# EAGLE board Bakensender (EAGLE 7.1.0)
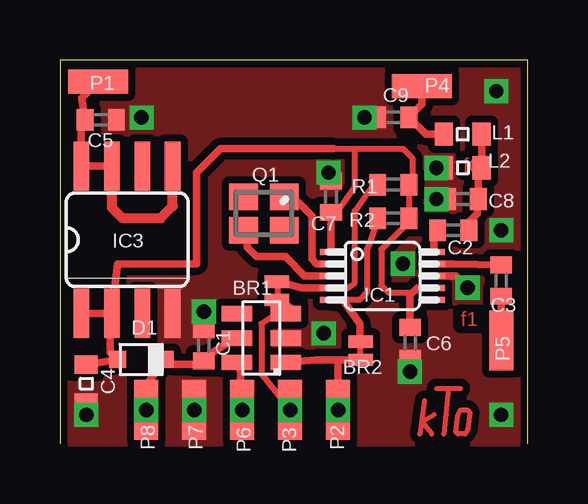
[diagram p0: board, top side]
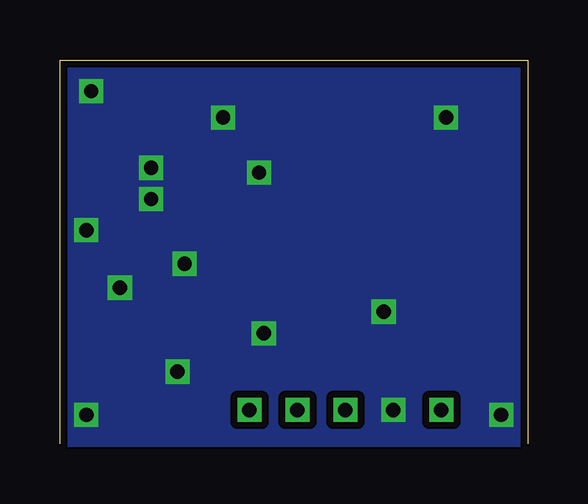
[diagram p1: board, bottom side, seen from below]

Size 19.5 x 16 mm. Coordinates in mm from the lower left corner, seen from the top.
Outline: 19.5,0 19.5,16 0,16 0,0
Copper layers (1*16): Top 0.035mm / dielectric 0.5mm / Bottom 0.035mm
Design rules "default *": minimum track width 10mil, minimum drill 0.6mm, track to track 8mil, track to pad 8mil, pad to pad 8mil, via to via 8mil, smd to smd 8mil, copper to edge 4mil, drill to drill 8mil, minimum pad ring 10mil, minimum via ring 8mil, stop-mask expansion 4mil, vias tented up to drill 0mil, thermal gap 10mil

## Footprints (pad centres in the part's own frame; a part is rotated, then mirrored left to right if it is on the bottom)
0402 = smd 0.7 x 0.9: 1 -0.65,0; 2 0.65,0
0603 = smd 0.762 x 0.965: 1 -0.787,0; 2 0.787,0
SOD323_S = smd 0.7 x 0.7: P$1 -0.997,-0.005; P$2 0.997,-0.005
MSOP10 = smd 0.25 x 0.9: 1 0,0; 2 0.5,0; 3 1,0; 4 1.5,0; 5 2,0; 6 2,4.3; 7 1.5,4.3; 8 1,4.3; 9 0.5,4.3; 10 0,4.3
SOT23-6 = smd 0.635 x 1.27: 1 -1.016,-1.016; 2 0,-1.016; 3 1.016,-1.016; 4 1.016,1.016; 5 0,1.016; 6 -1.016,1.016
SO08 = smd 0.66 x 2.032: 1 -1.905,-3.073; 2 -0.635,-3.073; 3 0.635,-3.073; 4 1.905,-3.073; 5 1.905,3.073; 6 0.635,3.073; 7 -0.635,3.073; 8 -1.905,3.073
ANSCHL7 = smd 2.5 x 1: P$1 0,0
FA-20H = smd 1.2 x 1.1: 1 -0.85,-0.7; 2 0.85,-0.7; 3 0.85,0.7; 4 -0.85,0.7
SMDJUMP = smd 1.016 x 0.508: P$1 0.051,0.508; P$2 0.051,-0.254

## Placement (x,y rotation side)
C1  100n  [0402]  6,4.1 90 top
C2  10n  [0402]  16.4,8.9 180 top
C3  10n  [0402]  18.4,6.8 90 top
C4  1u/6V  [0603]  1.1,2.5 90 top
C5  100n  [0402]  1.7,13.5 180 top
C6  100n  [0402]  14.6,4.2 90 top
C7  100n  [0402]  11.3,10.3 90 top
C8  39p  [0402]  16.8,10.2 0 top
C9  39p  [0402]  13.9,13.6 0 top
D1  BAT 62-03W  [SOD323_S]  3.4,3.5 180 top
IC1  SI5351A  [MSOP10]  11.3,8 270 top
IC2  PIC10F206  [SOT23-6]  8.4,4.4 90 top
IC3  MIC5200  [SO08]  2.8,8.5 0 top
L1  47nH  [0603]  16.8,12.9 180 top
L2  entfällt  [0603]  16.8,11.5 0 top
P1  +Ub  [ANSCHL7]  1.6,15.1 180 top
P2  Clk  [ANSCHL7]  11.6,1.4 270 top
P3  Data  [ANSCHL7]  9.6,1.4 270 top
P4  f0  [ANSCHL7]  15.1,14.9 0 top
P5  f1  [ANSCHL7]  18.4,4.3 270 top
P6  MCLR  [ANSCHL7]  7.6,1.4 270 top
P7  GND  [ANSCHL7]  5.6,1.4 270 top
P8  3V3  [ANSCHL7]  3.6,1.4 270 top
Q1  40MHz  [FA-20H]  8.5,9.6 180 top
R1  4k7  [0402]  13.9,10.8 0 top
R2  4k7  [0402]  13.9,9.4 0 top
U$9  SMDJUMP  [SMDJUMP]  12.6,4 180 top
U$10  SMDJUMP  [SMDJUMP]  9.1,6.5 180 top
U$11  [KTO]  15.6,1.1 0 top

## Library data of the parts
C1-C9 D1 IC3 R1 R2 = otto
IC1 = otto_afu
IC2 = microchip-3
L1 L2 P1-P8 U$9-U$11 = otto_L
Q1 = crystal

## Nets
GND: C1.2 C4.1 C5.1 C6.1 C7.2 C8.1 C9.1 IC1.8 IC2.2 IC3.4 L2.1 P7.P$1
N$1: IC2.1 P2.P$1 U$9.P$1
N$2: IC2.3 P3.P$1 U$10.P$1
N$3: IC1.3 Q1.3
N$4: IC1.2 Q1.1
N$5: IC2.6 P6.P$1
N$7: C3.1 P5.P$1
N$8: IC1.5 R2.1 U$9.P$2
N$9: C5.2 IC3.5 IC3.7 IC3.8 P1.P$1
N$10: C3.2 IC1.9
N$11: C2.2 IC1.10
N$12: C4.2 C6.2 C7.1 D1.P$2 IC1.1 IC1.7 IC3.1 IC3.2 R1.2 R2.2
N$14: IC1.4 R1.1 U$10.P$2
N$15: C1.1 D1.P$1 IC2.5 P8.P$1
N$16: C2.1 C8.2 L1.1 L2.2
N$17: C9.2 L1.2 P4.P$1

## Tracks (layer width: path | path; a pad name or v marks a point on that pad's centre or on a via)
GND  (via drill 0.6)
  Top 0.305: IC1.8 16.5,7 v17,6.5
  other vias: 18.2,14.7 6,5.5 11.2,11.3 14.6,3 14.3,7.5 18.4,1.2 11,4.6 1.1,1.2 3.4,13.6 5.6,1.4 12.7,13.6 15.7,10.2 15.7,11.5 18.4,8.9
  pour Top (isolate 0.305, no thermals): 0,16 19.5,16 19.5,0 0,0
  pour Bottom (isolate 0.305, no thermals): 0,16 19.5,16 19.5,0 0,0
N$1  (via drill 0.6)
  Top 0.305: IC2.1 10.7,3.48 11.6,3.48 | 11.6,3.48 12.3,3.48 12.31,3.49 U$9.P$1 | P2.P$1 11.6,3.48
  other vias: 11.6,1.4
N$2  (via drill 0.6)
  Top 0.254: 9.8,5.53 9.23,5.53 8.4,5 8.4,2.9 P3.P$1
  Top 0.305: IC2.3 9.8,5.53 9.89,5.53 U$10.P$1
  other vias: 9.6,1.4
N$3
  Top 0.305: IC1.3 10.2,7 9.4,7.8 8.2,7.8 7.8,8.2 7.8,8.75 Q1.3
N$4
  Top 0.305: IC1.2 10.7,7.5 10.5,7.7 10.5,9.5 9.9,10.1 9.55,10.1 Q1.1
N$5  (via drill 0.6)
  Top 0.305: P6.P$1 7.5,3.2 IC2.6
  other vias: 7.6,1.4
N$6
  Top 0.254: 12.5,4.2 12.5,3.6
N$7
  Top 0.305: C3.1 P5.P$1
N$8
  Top 0.254: R2.1 13.05,8.75 12.8,8.1 12.8,6.3 12.5,6 IC1.5
  Top 0.305: IC1.5 11.8,6 12.5,5 12.5,4.3 U$9.P$2
N$9
  Top 0.305: P1.P$1 0.91,14.41 C5.2 0.9,13.48 IC3.8 IC3.7
  Top 0.406: IC3.7 2.17,9.84 2.6,9.4 4.2,9.4 4.7,9.9 4.7,11.27 IC3.5
N$10
  Top 0.305: IC1.9 16.41,7.5 C3.2
N$11
  Top 0.305: IC1.10 15.6,8.79 C2.2
N$12
  Top 0.254: 11.4,12.3 12.3,12.3 | 12.3,12.3 14.3,12.3 14.7,11.9 14.7,10.65 R1.2 R2.2 14.5,9.2 13.4,8.1 13.4,6.6 13.7,6.3 14.5,6.3 14.6,6.2 14.65,6.25 | C7.1 11.35,9.35 12.3,10.7 12.3,12.3
  Top 0.305: 2.1,5.1 2.4,7.5 5.7,7.5 5.7,11.3 6.7,12.3 11.4,12.3 | IC1.1 C7.1 11.21,9.5 | C6.2 14.6,5.1 | IC1.7 14.9,6.5 14.6,6.2 14.6,5.1 | 14.6,5.1 14.5,5 | IC3.1 IC3.2 2.14,5.1 2.1,5.1 | C4.2 2.32,3.49 D1.P$2 2.1,3.81 2.1,5.1
N$14
  Top 0.254: IC1.4 12,6.5 12.3,6.7 12.3,9.7 13.2,11 R1.1
  Top 0.305: IC1.4 10.1,6.5 U$10.P$2
N$15  (via drill 0.6)
  Top 0.305: IC2.5 7.3,4.4 5.9,3.5 6.1,3.39 C1.1 5.85,3.3 4.8,3.3 4.61,3.4 D1.P$1 3.5,2.3 3.6,2.2 P8.P$1
  other vias: 3.6,1.4
N$16
  Top 0.305: C2.1 17.05,9.25 17.4,9.6 17.4,10.15 C8.2 17.45,11.36 L2.2 L1.1
N$17
  Top 0.305: L1.2 15.25,12.9 C9.2 15.1,14.15 P4.P$1
N$18
  Top 0.254: 9.1,6.1 9.1,6.6

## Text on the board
Top: f0 | f1
tPlace: BR1 | BR2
